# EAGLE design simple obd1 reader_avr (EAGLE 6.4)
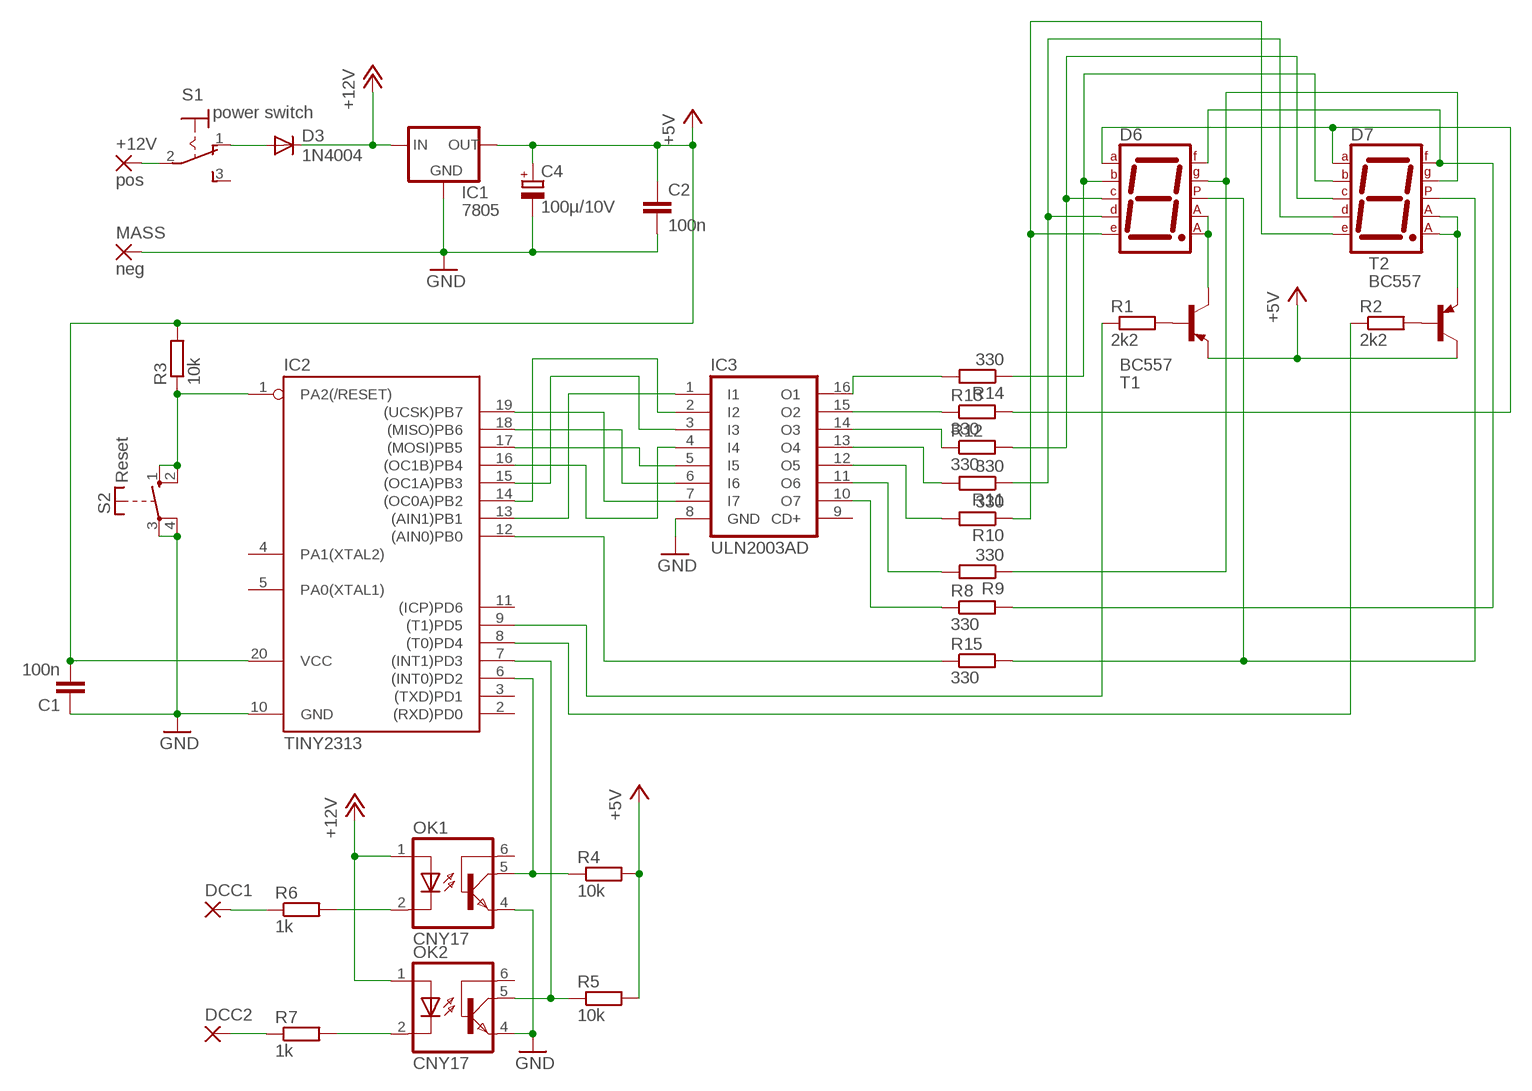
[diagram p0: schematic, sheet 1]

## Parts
+12V  pos  2,15/1,0  [2,15/1,0]
C1  100n  C-EU025_050-025X075  [C025_050-025X075]
C2  100n  C-EU025_050-025X075  [C025_050-025X075]
C4  100µ/10V  CPOL-EUE2.5-7  [E2,5-7]
D3  1N4004  [DO41-10]
D6  7SEG-CA  [7SEG-13]
D7  7SEG-CA  [7SEG-13]
DCC1  2,15/1,0  [2,15/1,0]
DCC2  2,15/1,0  [2,15/1,0]
IC1  7805  78XXL  [78XXL]
IC2  TINY2313  TINY2313-*P*  [DIL20]
IC3  ULN2003AD  [SO16]
MASS  neg  2,15/1,0  [2,15/1,0]
OK1  CNY17  [DIL06]
OK2  CNY17  [DIL06]
R1  2k2  R-EU_0207/7  [0207/7]
R2  2k2  R-EU_0207/7  [0207/7]
R3  10k  R-EU_0207/7  [0207/7]
R4  10k  R-EU_0207/7  [0207/7]
R5  10k  R-EU_0207/7  [0207/7]
R6  1k  R-EU_0207/7  [0207/7]
R7  1k  R-EU_0207/7  [0207/7]
R8  330  R-EU_0207/2V  [0207/2V]
R9  330  R-EU_0207/2V  [0207/2V]
R10  330  R-EU_0207/7  [0207/7]
R11  330  R-EU_0207/2V  [0207/2V]
R12  330  R-EU_0207/7  [0207/7]
R13  330  R-EU_0207/7  [0207/7]
R14  330  R-EU_0207/7  [0207/7]
R15  330  R-EU_0207/7  [0207/7]
S1  power switch  M9040P  [M9040P]
S2  Reset  DTE6K  [DTE6K]
T1  BC557  [TO92-EBC]
T2  BC557  [TO92-EBC]

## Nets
+5V: C1.2 C2.1 C4.+ IC1.OUT IC2.20(VCC) R3.2 R4.2 R5.2 T1.E T2.C
+12V: D3.C IC1.IN OK1.1(A) OK2.1(A)
GND: C1.1 C2.2 C4.- IC1.GND IC2.10(GND) IC3.8(GND) MASS.1(P) OK1.4(EMI) OK2.4(EMI) S2.3(P) S2.4(P)
N$1: D6.5(DP) D7.5(DP) R15.2
N$2: D6.3(CA1) D6.8(CA2) T1.C
N$3: IC2.12((AIN0)PB0) R15.1
N$4: D6.2(D) D7.2(D) R11.1
N$5: D7.3(CA1) D7.8(CA2) T2.E
N$6: IC3.16(O1) R14.2
N$7: R1.2 T1.B
N$8: R2.2 T2.B
N$9: IC2.9((T1)PD5) R1.1
N$10: IC2.7((INT1)PD3) OK2.5(COL) R5.1
N$11: IC3.15(O2) R13.1
N$12: IC3.14(O3) R12.1
N$13: IC3.13(O4) R11.2
N$14: IC3.12(O5) R10.2
N$15: IC3.11(O6) R9.2
N$16: IC3.10(O7) R8.1
N$17: IC2.13((AIN1)PB1) IC3.1(I1)
N$18: IC2.8((T0)PD4) R2.1
N$19: D6.7(A) D7.7(A) R13.2
N$20: D6.9(F) D7.9(F) R8.2
N$21: D6.10(G) D7.10(G) R9.1
N$22: IC2.19((UCSK)PB7) IC3.7(I7)
N$23: D6.6(B) D7.6(B) R14.1
N$24: D6.4(C) D7.4(C) R12.2
N$25: OK2.2(C) R7.2
N$26: D6.1(E) D7.1(E) R10.1
N$27: IC2.18((MISO)PB6) IC3.6(I6)
N$28: OK1.2(C) R6.2
N$29: IC2.17((MOSI)PB5) IC3.5(I5)
N$30: IC2.6((INT0)PD2) OK1.5(COL) R4.1
N$31: +12V.1(P) S1.2(P)
N$32: IC2.1(PA2(/RESET)) R3.1 S2.1(S) S2.2(S)
N$33: DCC1.1(P) R6.1
N$34: DCC2.1(P) R7.1
N$35: D3.A S1.1(O)
N$36: IC2.16((OC1B)PB4) IC3.4(I4)
N$37: IC2.15((OC1A)PB3) IC3.3(I3)
N$39: IC2.14((OC0A)PB2) IC3.2(I2)
Unconnected: IC2.2((RXD)PD0) IC2.3((TXD)PD1) IC2.4(PA1(XTAL2)) IC2.5(PA0(XTAL1)) IC2.11((ICP)PD6) IC3.9(CD+) OK1.6(BAS) OK2.6(BAS) S1.3(S)

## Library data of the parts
+12V DCC1 DCC2 MASS = wirepad:2,15/1,0: THROUGH-HOLE PAD
C1 C2 = rcl:C-EU: CAPACITOR, European symbol
C4 = rcl:CPOL-EU: POLARIZED CAPACITOR, European symbol
D3 = diode:1N4004: DIODE
D6 D7 = special:7SEG-CA: 7-segment DISPLAY single anode, 13 mm
IC1 = v-reg:78XXL: VOLTAGE REGULATOR
IC2 = avr-7:TINY2313*: Atmel Tiny2313 2K Flash, 128 bytes EEPROM, 128 bytes RAM
IC3 = uln-udn:ULN2003A: DRIVER ARRAY
OK1 OK2 = optocoupler:CNY17: SIEMENS OPTO COUPLER; MPN: CNY17-1; OC_FARNELL: 1045399; OC_NEWARK: 05M4044
R1-R15 = rcl:R-EU_: RESISTOR, European symbol
S1 = switch:M9040P: TOGGLE SWITCH Marquardt
S2 = switch-misc:DT: ITT SWITCH
T1 T2 = transistor-pnp:BC557*: PNP Transistror

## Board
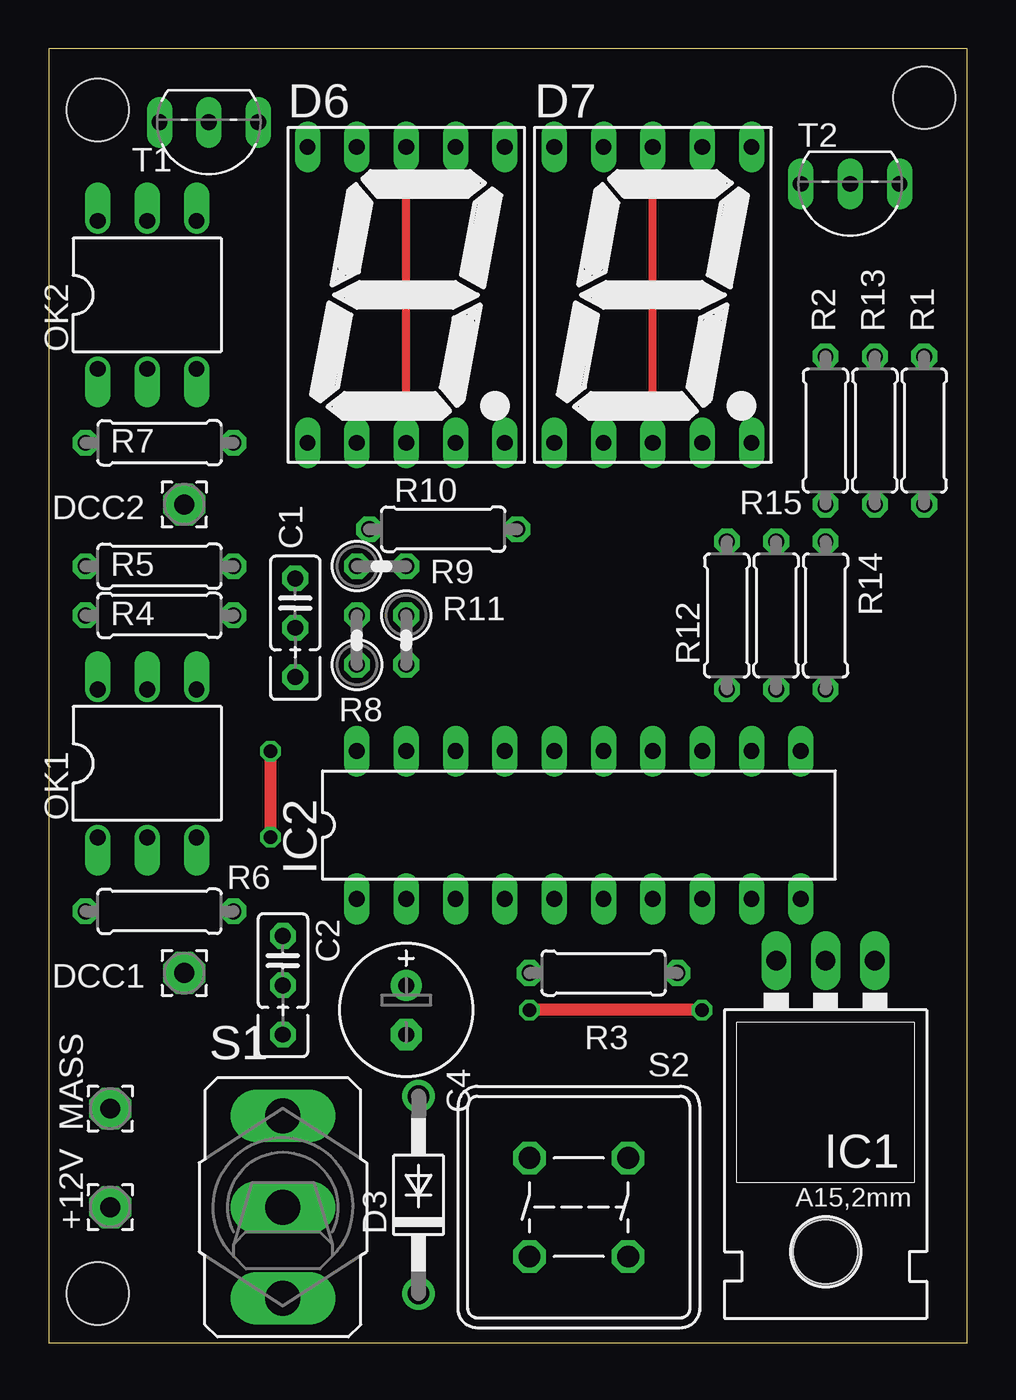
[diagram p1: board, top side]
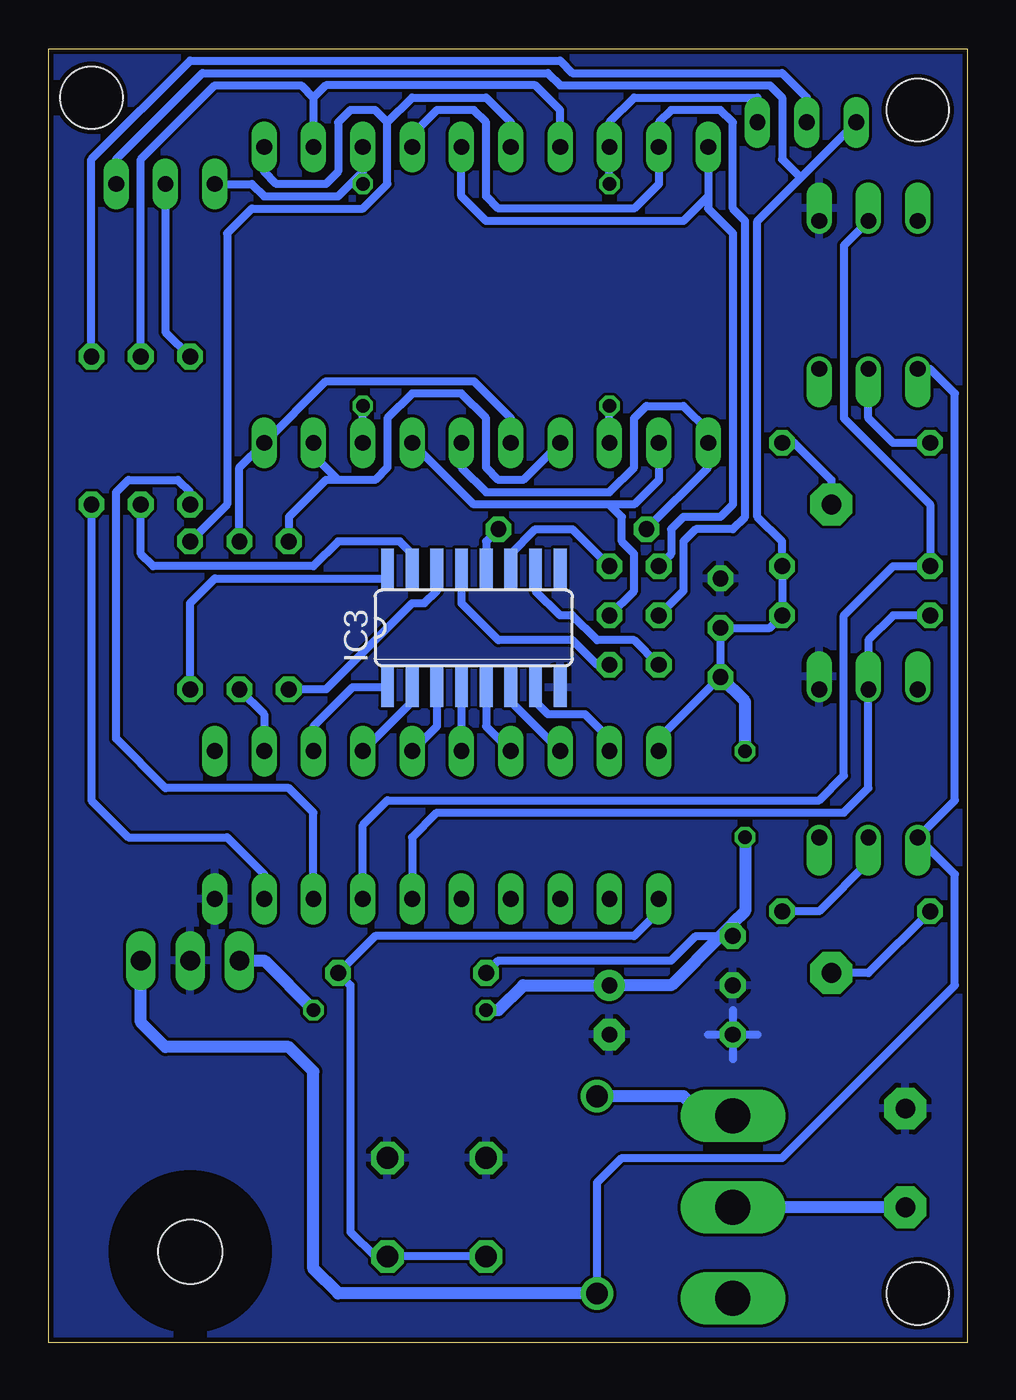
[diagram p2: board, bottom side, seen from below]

Size 47.3 x 66.67 mm. Coordinates in mm from the lower left corner, seen from the top.
Outline: 0,0 47.3,0 47.3,66.67 0,66.67 0,0
Copper layers (1*16): Top 0.035mm / dielectric 1.5mm / Bottom 0.035mm
Design rules "default": minimum track width 6mil, minimum drill 12mil, track to track 6mil, track to pad 6mil, pad to pad 6mil, via to via 6mil, smd to smd 0mil, copper to edge 10mil, drill to drill 10mil, minimum pad ring 10mil, minimum via ring 6mil, stop-mask expansion 2mil, vias tented up to drill 100mil, thermal gap 10mil
Holes 3.2 mm at 45.09,64.14 2.54,2.54 2.54,63.5

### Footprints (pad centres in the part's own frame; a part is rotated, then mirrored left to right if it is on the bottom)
2,15/1,0 = drill 1.016 pad 2.159 octagon: 1 0,0
C025_050-025X075 = drill 0.813 octagon: 1 -1.27,0; 2 1.27,0; 3 3.81,0
E2,5-7 = drill 0.813 pad 1.6: + -1.27,0 | drill 0.813 pad 1.6 octagon: - 1.27,0
DO41-10 = drill 1.118: A 5.08,0; C -5.08,0
7SEG-13 = drill 0.813 long: 1 -5.08,-7.62; 2 -2.54,-7.62; 3 0,-7.62; 4 2.54,-7.62; 5 5.08,-7.62; 6 5.08,7.62; 7 2.54,7.62; 8 0,7.62; 9 -2.54,7.62; 10 -5.08,7.62
78XXL = drill 1.016 long: GND 0,-3.81; IN -2.54,-3.81; OUT 2.54,-3.81 | hole 3.302: 0,11.176
DIL20 = drill 0.813 long: 1 -11.43,-3.81; 2 -8.89,-3.81; 3 -6.35,-3.81; 4 -3.81,-3.81; 5 -1.27,-3.81; 6 1.27,-3.81; 7 3.81,-3.81; 8 6.35,-3.81; 9 8.89,-3.81; 10 11.43,-3.81; 11 11.43,3.81; 12 8.89,3.81; 13 6.35,3.81; 14 3.81,3.81; 15 1.27,3.81; 16 -1.27,3.81; 17 -3.81,3.81; 18 -6.35,3.81; 19 -8.89,3.81; 20 -11.43,3.81
SO16 = smd 0.66 x 2.032: 1 -4.445,-3.073; 2 -3.175,-3.073; 3 -1.905,-3.073; 4 -0.635,-3.073; 5 0.635,-3.073; 6 1.905,-3.073; 7 3.175,-3.073; 8 4.445,-3.073; 9 4.445,3.073; 10 3.175,3.073; 11 1.905,3.073; 12 0.635,3.073; 13 -0.635,3.073; 14 -1.905,3.073; 15 -3.175,3.073; 16 -4.445,3.073
DIL06 = drill 0.813 offset: 1 -2.54,-3.81; 2 0,-3.81; 3 2.54,-3.81; 4 2.54,3.81; 5 0,3.81; 6 -2.54,3.81
0207/7 = drill 0.813 octagon: 1 -3.81,0; 2 3.81,0
0207/2V = drill 0.813 octagon: 1 -1.27,0; 2 1.27,0
M9040P = drill 1.803 long: 1 0,4.699; 2 0,0; 3 0,-4.699
DTE6K = drill 1.118 octagon: 1 -2.54,2.54; 2 2.54,2.54; 3 2.54,-2.54; 4 -2.54,-2.54
TO92-EBC = drill 0.813 long: B 0,-1.27; C -2.54,-1.27; E 2.54,-1.27

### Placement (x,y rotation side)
+12V  3.17,6.99 90 top
C1  12.7,38.1 270 top
C2  12.06,19.68 270 top
C4  18.41,17.14 270 top
D3  19.05,7.62 90 top
D6  18.41,53.98 0 top
D7  31.11,53.98 0 top
DCC1  6.99,19.05 90 top
DCC2  6.99,43.18 90 top
IC1  40.01,15.88 180 top
IC2  27.3,26.67 0 top
IC3  25.4,36.83 0 bottom
MASS  3.17,12.06 90 top
OK1  5.08,29.84 0 top
OK2  5.08,53.98 0 top
R1  45.09,46.99 90 top
R2  40.01,46.99 90 top
R3  28.57,19.05 180 top
R4  5.71,37.47 0 top
R5  5.71,40.01 0 top
R6  5.71,22.23 0 top
R7  5.71,46.35 180 top
R8  15.88,36.2 90 top
R9  17.14,40.01 0 top
R10  20.32,41.91 0 top
R11  18.41,36.2 270 top
R12  34.92,37.47 90 top
R13  42.55,46.99 90 top
R14  40.01,37.47 270 top
R15  37.47,37.47 90 top
S1  12.06,6.99 0 top
S2  27.3,6.99 180 top
T1  8.26,61.59 180 top
T2  41.27,58.42 180 top

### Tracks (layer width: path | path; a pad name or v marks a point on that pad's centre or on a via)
+5V  (via drill 0.7)
  Top 0.61: v11.43,26.04 v11.43,30.48 | v33.66,17.14 v24.77,17.14
  Bottom 0.406: IC2.20 15.88,31.11 12.7,34.29 C1.2 10.16,36.83 R4.2 R5.2 9.53,41.27 10.79,42.55 10.79,57.78 8.57,60.01 | R3.2 24.13,19.68 15.24,19.68 13.97,20.95 12.7,20.95 | C2.1 12.06,21.59 | 8.57,60.01 T1.E | T2.C 43.81,60.96 39.37,65.41 21.59,65.41 20.95,64.77 10.16,64.77 9.53,64.14 9.53,60.96 8.57,60.01
  Bottom 0.61: v11.43,30.48 11.43,33.02 12.7,34.29 | IC1.OUT 36.2,19.68 v33.66,17.14 | v24.77,17.14 24.13,17.14 22.86,18.41 C4.+ 15.24,18.41 12.7,20.95 12.06,21.59 11.43,22.23 v11.43,26.04
+12V
  Bottom 0.406: D3.C 19.05,8.26 17.78,9.53 9.53,9.53 0.64,18.41 0.64,24.13 OK1.1 0.64,27.94 0.64,48.9 1.91,50.16 OK2.1
  Bottom 0.61: D3.C 32.38,2.54 33.66,3.81 33.66,13.97 34.92,15.24 41.27,15.24 42.55,16.51 IC1.IN
GND
  Bottom 0.406: 12.06,17.14 12.06,14.61 | 13.34,15.88 10.79,15.88
  pour Bottom: 0,66.67 0,0 47.62,0 47.62,66.67
N$1
  Bottom 0.406: D6.5 23.5,47.62 25.4,49.53 33.02,49.53 D7.5 37.47,45.09 R15.2
N$2  (via drill 0.7)
  Top 0.406: v18.41,48.26 v18.41,59.69
  Bottom 0.406: D6.3 v18.41,48.26 | v18.41,59.69 D6.8 18.41,62.87 17.14,64.14 10.79,64.14 T1.C
N$3
  Bottom 0.406: R15.1 36.2,32.38 IC2.12
N$4
  Bottom 0.406: D6.2 15.88,44.45 17.14,43.18 18.41,43.18 | D7.2 25.4,43.18 18.41,43.18 | R11.1 17.14,38.73 17.14,40.64 17.78,41.27 17.78,42.55 18.41,43.18
N$5  (via drill 0.7)
  Top 0.406: v31.11,48.26 v31.11,59.69
  Bottom 0.406: 31.11,60.33 32.38,59.05 36.2,59.05 36.83,59.69 T2.E | 31.11,60.33 D7.8 | D7.3 v31.11,48.26 | v31.11,59.69 31.11,60.33
N$6
  Bottom 0.406: IC3.16 29.84,39.37 38.73,39.37 40.01,38.1 R14.2
N$7
  Bottom 0.406: R1.2 45.09,60.96 40.01,66.04 20.95,66.04 20.32,65.41 9.53,65.41 8.26,64.14 T1.B
N$8
  Bottom 0.406: T2.B 41.27,52.07 R2.2
N$9
  Bottom 0.406: IC2.9 36.2,24.13 38.1,26.04 43.18,26.04 45.09,27.94 R1.1
N$10
  Bottom 0.406: IC2.7 31.11,26.67 29.84,27.94 7.62,27.94 6.35,29.21 6.35,37.47 3.81,40.01 R5.1 1.91,43.18 6.35,47.62 6.35,56.52 OK2.5
N$11
  Bottom 0.406: IC3.15 28.57,40.64 29.21,41.27 32.38,41.27 33.66,40.01 41.91,40.01 42.55,40.64 R13.1
N$12
  Bottom 0.406: R12.1 33.02,33.66 28.57,38.1 27.94,38.1 27.3,38.73 IC3.14
N$13
  Bottom 0.406: R11.2 19.05,34.92 20.32,36.2 24.13,36.2 26.04,38.1 IC3.13
N$14
  Bottom 0.406: R10.2 24.77,41.27 IC3.12
N$15
  Bottom 0.406: IC3.11 23.5,40.64 22.23,41.91 20.32,41.91 R9.2
N$16
  Bottom 0.406: R8.1 17.14,36.2 19.05,36.2 20.32,37.47 20.95,37.47 22.23,38.73 IC3.10
N$17
  Bottom 0.406: IC3.1 31.65,33.76 33.66,31.75 IC2.13
N$18
  Bottom 0.406: IC2.8 33.66,27.3 34.92,28.57 41.27,28.57 43.81,31.11 43.81,43.81 43.18,44.45 40.64,44.45 40.01,43.81 R2.1
N$19
  Bottom 0.406: D6.7 20.95,63.5 22.23,64.77 33.02,64.77 33.66,64.14 | 33.66,64.14 D7.7 | R13.2 42.55,60.96 38.73,64.77 34.29,64.77 33.66,64.14
N$20
  Bottom 0.406: D7.9 28.57,62.23 27.3,63.5 25.4,63.5 24.77,62.87 24.77,59.05 24.13,58.42 17.14,58.42 15.88,59.69 D6.9 15.88,62.87 15.24,63.5 12.7,63.5 12.06,62.87 12.06,58.42 11.43,57.78 11.43,42.55 12.06,41.91 13.97,41.91 14.61,41.27 14.61,38.73 R8.2
N$21
  Bottom 0.406: 13.34,59.05 14.61,57.78 24.77,57.78 26.04,59.05 D7.10 | D6.10 13.34,59.05 | R9.1 15.24,40.64 15.24,41.91 14.61,42.55 12.7,42.55 12.06,43.18 12.06,57.15 13.34,58.42 13.34,59.05
N$22
  Bottom 0.406: IC3.7 22.23,33.02 21.59,32.38 19.68,32.38 18.41,31.11 IC2.19
N$23
  Bottom 0.406: D6.6 23.5,62.87 24.77,64.14 28.57,64.14 29.84,62.87 | D7.6 36.2,60.33 35.56,59.69 33.02,59.69 32.38,60.33 32.38,62.87 31.75,63.5 30.48,63.5 29.84,62.87 | 29.84,62.87 29.84,59.69 31.11,58.42 36.83,58.42 38.1,57.15 38.1,43.18 R14.1
N$24
  Bottom 0.406: D6.4 22.86,44.45 24.13,44.45 24.77,45.09 24.77,47.62 26.04,48.9 28.57,48.9 29.84,47.62 29.84,45.09 30.48,44.45 32.38,44.45 | D7.4 33.66,45.72 32.38,44.45 | 32.38,44.45 33.02,44.45 34.92,42.55 R12.2
N$25
  Bottom 0.406: R7.2 3.81,46.35 5.08,47.62 OK2.2
N$26
  Bottom 0.406: D7.1 26.04,45.09 24.77,43.81 18.41,43.81 17.14,45.09 17.14,47.62 16.51,48.26 14.61,48.26 13.34,46.99 D6.1 13.34,45.09 R10.1
N$27
  Bottom 0.406: IC3.6 23.5,33.02 IC2.18
N$28
  Bottom 0.406: OK1.2 5.08,24.77 7.62,22.23 R6.2
N$29
  Bottom 0.406: IC3.5 24.77,31.75 IC2.17
N$30
  Bottom 0.406: R4.1 3.81,37.47 5.08,36.2 OK1.5 5.08,28.57 6.35,27.3 27.3,27.3 28.57,26.04 IC2.6
N$31
  Bottom 0.61: +12V.1 S1.2
N$32
  Bottom 0.406: S2.2 S2.1 30.48,4.45 31.75,5.71 31.75,18.41 R3.1 30.48,20.95 17.14,20.95 15.88,22.23 IC2.1
N$33
  Bottom 0.406: R6.1 5.08,19.05 DCC1.1
N$34
  Bottom 0.406: R7.1 8.89,46.35 6.99,44.45 DCC2.1
N$35
  Bottom 0.61: S1.1 13.59,11.68 14.61,12.7 D3.A
N$36
  Bottom 0.406: IC3.4 IC2.16
N$37
  Bottom 0.406: IC3.3 27.3,31.75 IC2.15
N$39
  Bottom 0.406: IC3.2 28.57,33.02 IC2.14

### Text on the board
bRestrict: RX7 EPCR v1 | cd-pc.mazda-club.be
